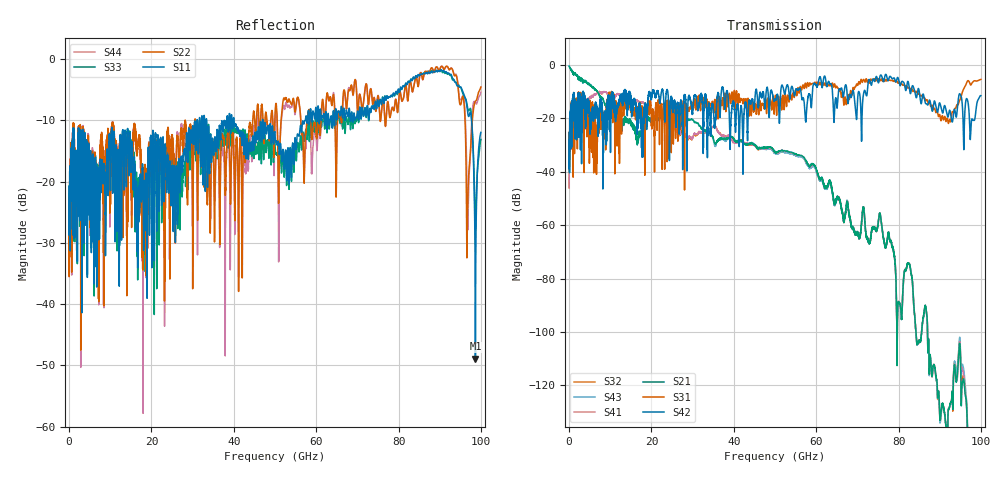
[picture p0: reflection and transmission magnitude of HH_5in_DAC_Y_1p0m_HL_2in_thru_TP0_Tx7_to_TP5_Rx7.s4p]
# GHz S RI R 45
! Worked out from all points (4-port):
!   4000 points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, 25 MHz to 100 GHz, reference 45 ohm
!   strongest paths, dB at 25 MHz, 25.02 GHz, 50.02 GHz, 75.03 GHz, 100 GHz:
!     S42: -38.8, -15.0, -12.9, -6.4, -11.5
!     S31: -39.0, -14.4, -12.1, -5.7, -5.4
!     S21: -0.5, -19.9, -32.5, -59.5, -182.2
!     S41: -46.0, -22.0, -32.6, -59.5, -184.1
!     S43: -0.5, -20.1, -32.9, -59.5, -176.6
!     S32: -46.0, -22.2, -32.7, -59.5, -183.3
!   lowest |S11| = -48.9 dB at 98.67 GHz (marker M1), VSWR 1.01, Z = 45.3 + j0.0119 ohm
!   |S11| at or under -10 dB: start of sweep to 31.06 GHz; 40.08 GHz to 46.97 GHz (6.89 GHz wide, 15.8 % of centre); 47.06 GHz to 57.36 GHz (10.3 GHz wide, 19.7 % of centre)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
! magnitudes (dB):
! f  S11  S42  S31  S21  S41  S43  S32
! 25 MHz  -23.1  -38.8  -39.0  -0.5  -46.0  -0.5  -46.0
! 2.125 GHz  -18.3  -15.1  -15.5  -4.6  -13.4  -4.6  -13.4
! 11.9 GHz  -17.9  -15.7  -18.4  -21.6  -10.8  -21.6  -10.8
! 56.52 GHz  -11.7  -12.7  -9.2  -34.0  -34.1  -34.7  -34.5
! 90.65 GHz  -2.0  -17.9  -19.0  -126.7  -126.8  -126.9  -126.8
! 98.67 GHz  -48.9  -18.7  -6.0  -159.0  -158.3  -155.6  -154.4
! 100 GHz  -12.0  -11.5  -5.4  -182.2  -184.1  -176.6  -183.3
